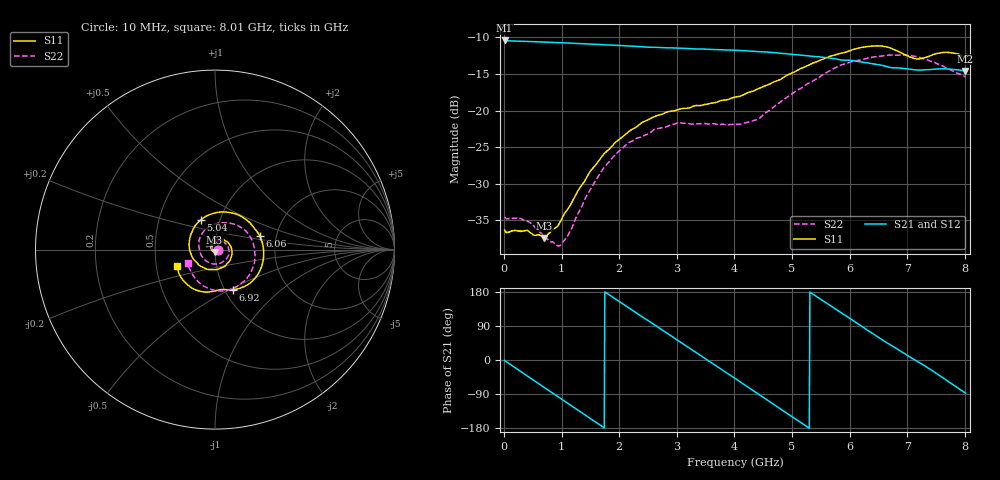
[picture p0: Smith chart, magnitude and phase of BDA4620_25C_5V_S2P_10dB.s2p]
!Agilent Technologies,E5071B,MY42404982,A.09.10
!Date: Wed May 06 09:00:15 2026
!Data & Calibration Information:
!Freq	S11:SOLT2(ON)	S21:SOLT2(ON)	S12:SOLT2(ON)	S22:SOLT2(ON)
# Hz S RI R 50
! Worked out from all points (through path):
!   801 points, 10 MHz to 8.01 GHz, reference 50 ohm
!   highest |S21| = -10.43 dB at 10 MHz (marker M1); lowest = -14.6 dB at 8.01 GHz (marker M2)
!   group delay of S21, straight-line fit = 280 ps
!   lowest |S11| = -37.4 dB at 700 MHz (marker M3), VSWR 1.03, Z = 49.8 - j1.33 ohm
!   |S11| at or under -10 dB: start of sweep to end of sweep
!   |S22| runs from -38.5 to -12.4 dB; largest |S21 - S12| = 0.0015
!   S11 on the Smith chart (normalised r, x): 10 MHz: 1.03, -0.00; 5.04 GHz: 0.81, +0.28; 6.06 GHz: 1.64, +0.26; 6.92 GHz: 1.09, -0.52; 8.01 GHz: 0.64, -0.12
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1e7  0.0152 -0.00108  0.3007 -0.00643  0.3011 -0.00656  0.0187 -0.00112
4.2e8  0.00966 -0.0115  0.2133 -0.205  0.2135 -0.2056  0.0135 -0.0109
7e8  -0.00213 -0.0133  0.0871 -0.2801  0.087 -0.2805  0.00315 -0.0136
9.8e8  -0.0166 -0.00564  -0.058 -0.2845  -0.0582 -0.2849  -0.00953 -0.00735
1.35e9  -0.0235 0.0203  -0.2174 -0.1861  -0.2177 -0.1863  -0.0169 0.0143
1.94e9  0.0185 0.058  -0.2628 0.0927  -0.2633 0.093  0.0143 0.0484
2.32e9  0.0635 0.046  -0.1449 0.2322  -0.1452 0.2325  0.0505 0.041
2.68e9  0.093 0.00332  0.0189 0.2688  0.0193 0.2692  0.0743 0.0121
2.99e9  0.0885 -0.0479  0.154 0.2184  0.1546 0.2184  0.0779 -0.0249
3.39e9  0.0403 -0.1002  0.2546 0.066  0.2552 0.0656  0.0447 -0.0676
4.01e9  -0.0854 -0.089  0.1708 -0.193  0.171 -0.1935  -0.0507 -0.0628
4.5e9  -0.1442 0.0203  -0.0372 -0.2492  -0.0373 -0.2497  -0.0912 0.0208
5.04e9  -0.0781 0.1657  -0.2164 -0.1075  -0.2168 -0.1075  -0.0284 0.1302
5.35e9  0.0219 0.2087  -0.2337 0.02  -0.2339 0.02  0.0513 0.1492
5.67e9  0.1412 0.1876  -0.1814 0.1377  -0.1814 0.1381  0.1381 0.1278
6.06e9  0.2498 0.0747  -0.0521 0.2123  -0.0522 0.2129  0.214 0.0317
6.37e9  0.2673 -0.0647  0.0621 0.2  0.0625 0.2001  0.2205 -0.0652
6.68e9  0.1913 -0.1897  0.1461 0.1332  0.1467 0.1334  0.1787 -0.1586
6.92e9  0.1004 -0.2235  0.1824 0.0664  0.1829 0.0664  0.1177 -0.2082
7.19e9  0.0295 -0.2229  0.1881 -0.0166  0.1887 -0.0167  0.0255 -0.2306
7.57e9  -0.0904 -0.2298  0.1439 -0.1287  0.1441 -0.1289  -0.086 -0.1857
8.01e9  -0.2112 -0.0888  0.0093 -0.1857  0.00931 -0.1863  -0.1521 -0.0751
